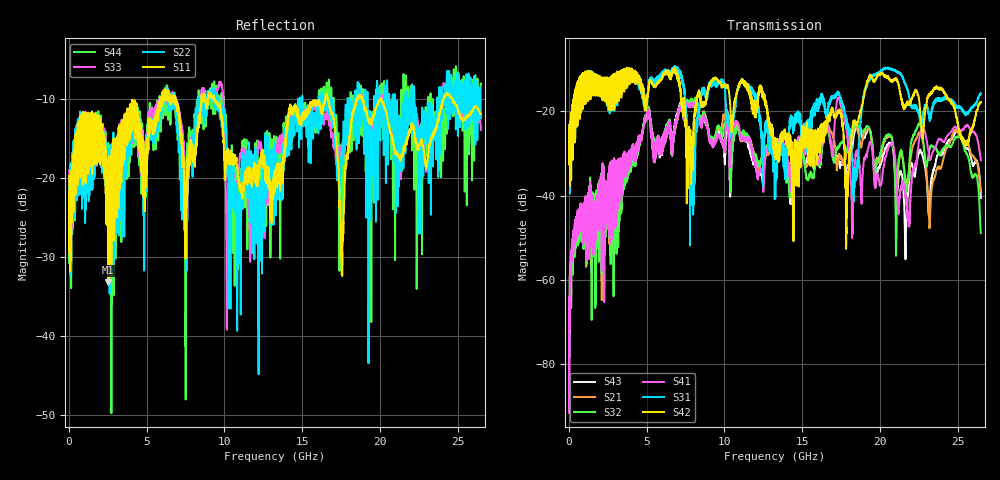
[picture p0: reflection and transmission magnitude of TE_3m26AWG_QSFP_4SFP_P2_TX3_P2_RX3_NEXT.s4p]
!Agilent Technologies,N5222A,MY51421691,A.10.00.00
!Agilent N5222A: A.10.00.00
!Date: Friday, January 30, 2015 12:35:55
!Correction: S11(Full 4 Port(1,2,3,4))
!S12(Full 4 Port(1,2,3,4))
!S13(Full 4 Port(1,2,3,4))
!S14(Full 4 Port(1,2,3,4))
!S21(Full 4 Port(1,2,3,4))
!S22(Full 4 Port(1,2,3,4))
!S23(Full 4 Port(1,2,3,4))
!S24(Full 4 Port(1,2,3,4))
!S31(Full 4 Port(1,2,3,4))
!S32(Full 4 Port(1,2,3,4))
!S33(Full 4 Port(1,2,3,4))
!S34(Full 4 Port(1,2,3,4))
!S41(Full 4 Port(1,2,3,4))
!S42(Full 4 Port(1,2,3,4))
!S43(Full 4 Port(1,2,3,4))
!S44(Full 4 Port(1,2,3,4))
!S4P File: Measurements: <S11,S12,S13,S14>,
!<S21,S22,S23,S24>,
!<S31,S32,S33,S34>,
!<S41,S42,S43,S44>:
# Hz S  dB  R 50.0
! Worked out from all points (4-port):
!   2650 points, 10 MHz to 26.5 GHz, reference 50 ohm
!   strongest paths, dB at 10 MHz, 6.63 GHz, 13.26 GHz, 19.88 GHz, 26.5 GHz:
!     S42: -25.1, -10.8, -28.8, -11.2, -17.8
!     S31: -24.9, -10.4, -34.1, -10.8, -15.7
!     S41: -68.3, -27.8, -29.2, -35.1, -31.6
!     S32: -67.5, -28.4, -30.5, -31.2, -48.9
!     S21: -68.7, -28.0, -31.1, -31.4, -38.9
!     S43: -69.1, -28.1, -31.0, -33.5, -40.6
!   lowest |S11| = -33.2 dB at 2.51 GHz (marker M1), VSWR 1.04, Z = 51 - j1.95 ohm
!   |S11| at or under -10 dB: start of sweep to 5.869 GHz; 9.354 GHz to 16.5 GHz (7.143 GHz wide, 55.3 % of centre); 20.09 GHz to 24.09 GHz (4.004 GHz wide, 18.1 % of centre)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
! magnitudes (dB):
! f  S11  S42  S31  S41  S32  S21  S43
! 10 MHz  -19.8  -25.1  -24.9  -68.3  -67.5  -68.7  -69.1
! 2.51 GHz  -33.2  -17.2  -19.7  -35.9  -36.8  -36.0  -36.7
! 6.96 GHz  -10.4  -12.3  -10.5  -21.3  -21.2  -21.8  -20.7
! 8.01 GHz  -16.5  -28.1  -30.9  -18.6  -17.4  -18.1  -17.9
! 21.66 GHz  -15.9  -18.5  -13.7  -39.9  -38.4  -36.1  -54.5
! 25.1 GHz  -11.9  -24.6  -19.2  -24.5  -26.0  -25.5  -25.0
! 26.5 GHz  -11.9  -17.8  -15.7  -31.6  -48.9  -38.9  -40.6
